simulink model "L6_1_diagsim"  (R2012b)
settings: Solver=ode45  SolverMode=SingleTasking  StartTime=0.0  StopTime=7  RelTol=1e-3
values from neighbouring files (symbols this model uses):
  A = [-1   0    [L6_1_diagonal.m]
  Ad = [-1 0    [L6_1_diagonal.m]
  B = [1; 0]    [L6_1_diagonal.m]
  Bd = V1*B    [L6_1_diagonal.m]
  C = [0 1]    [L6_1_diagonal.m]    (also in LinProb.m = LinProb(A.GetSize()))
  Cd = C*V    [L6_1_diagonal.m]
  D = 0    [L6_1_diagonal.m]    (also in V2_1_inverseZ.m = [1 -3 2]; V2_2_inverseZ.m = [1 0 0 0 0])

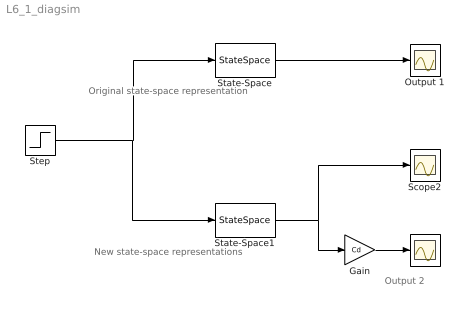
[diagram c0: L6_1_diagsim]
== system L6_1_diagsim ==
  note: New state-space representations
  note: Original state-space representation
  note: Output 2
  " " : Scope
  Gain : Gain  Gain=Cd  Multiplication=Matrix(K*u)
  Output 1 : Scope
  Scope2 : Scope
  State-Space : StateSpace  A=A  B=B  C=C  D=D  X0=0
  State-Space1 : StateSpace  A=Ad  B=Bd  C=eye(2)  D=[0; 0]  X0=0
  Step : Step  SampleTime=0
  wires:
  Step/1 -> State-Space1/1, State-Space/1
  State-Space/1 -> Output 1/1
  State-Space1/1 -> Gain/1, Scope2/1
  Gain/1 -> " "/1
